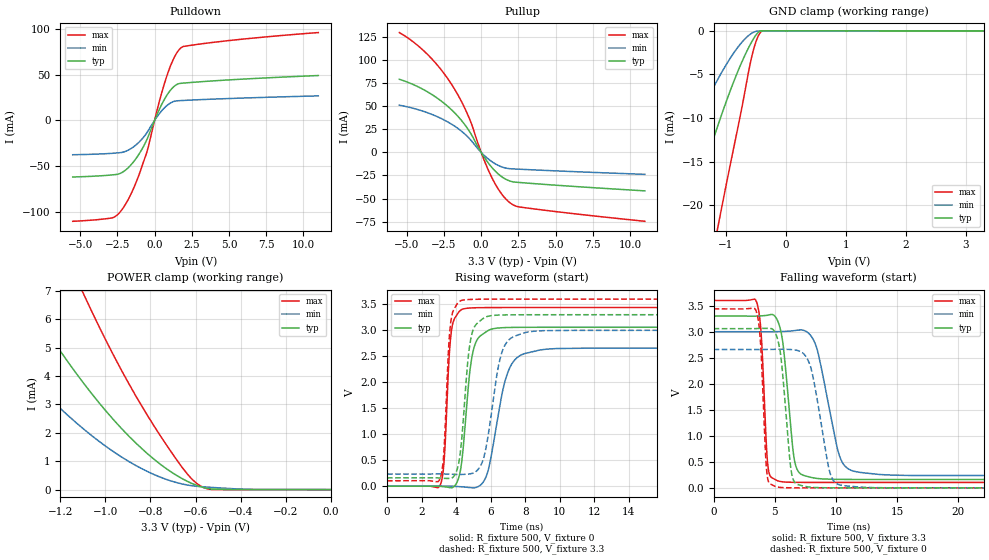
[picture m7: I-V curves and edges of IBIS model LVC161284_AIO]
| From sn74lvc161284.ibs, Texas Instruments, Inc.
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[Model]   LVC161284_AIO
Model_type  I/O
Vinl=0.8
Vinh=2.0
Enable   Active-Low
Vref =   0
Rref =   500
Cref =   50p
Vmeas =   1.5
| variable   typ   min   max
C_comp   7pF   NA   15pF
| C_pullup   4.48pF   2.95pF   5.26pF
| C_pulldown   4.78pF   2.73pF   7.37pF
| C_tri-state   3.06pF   2.68pF   3.49pF
[Temperature Range]   40   100   -40
| Ambient temperature   25   85   -40
[Voltage range]   3.3   3   3.6
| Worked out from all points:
|   slope of the pulldown table from 0 to 0.495 V, typ, clamps not added: 27.6 ohm
|   slope of the pullup table from 0 to 0.495 V, typ, clamps not added: 41.7 ohm
|   GND clamp passes 1 mA (typ) near -0.54 V on its own axis
|   POWER clamp passes 1 mA (typ) near -0.77 V on its own axis
|   rising waveform, R_fixture 500, V_fixture 0: 20-80 % time 523ps typ, 923ps min, 310ps max; typ from 0 V to 3.06 V
|   falling waveform, R_fixture 500, V_fixture 3.3: 20-80 % time 739ps typ, 1.41ns min, 417ps max; typ from 3.3 V to 0.161 V
|   rising waveform, R_fixture 500, V_fixture 3.3: 20-80 % time 482ps typ, 786ps min, 298ps max; typ from 0.161 V to 3.3 V
|   falling waveform, R_fixture 500, V_fixture 0: 20-80 % time 669ps typ, 1.16ns min, 393ps max; typ from 3.06 V to 0 V
[GND Clamp]
| LVC161284_AIO
|   Voltage   I(typ)   I(min)   I(max)
-5.5V     -124.6mA   -80.94mA   -210.5mA
-2.235V   -36.57mA   -22.18mA   -65.82mA
-1.66V    -22.55mA   -12.99mA   -42.47mA
-1.595V   -21.04mA   -12.01mA   -39.93mA
-1.35V    -15.52mA   -8.465mA   -30.56mA
-1.125V   -10.77mA   -5.487mA   -22.35mA
-1.095V   -10.16mA   -5.116mA   -21.29mA
-830mV    -5.215mA   -2.195mA   -12.23mA
-575mV    -1.378mA   -319uA     -3.275mA
-485mV    -388.3uA   -48.19uA   -1.058mA
-405mV    -426nA     -15.14uA   -79.63uA
3.3V      15.69pA    1.759uA    12.9pA
[POWER Clamp]
| LVC161284_AIO
|   Voltage   I(typ)   I(min)   I(max)
-5.5V     95.74mA    66.5mA     147.1mA
-1.67V    11.2mA     7.076mA    18.75mA
-1.63V    10.6mA     6.666mA    17.81mA
-1.375V   7.021mA    4.263mA    12.17mA
-1.34V    6.57mA     3.965mA    11.46mA
-1.095V   3.726mA    2.12mA     6.854mA
-960mV    2.424mA    1.312mA    4.669mA
-815mV    1.275mA    642.3uA    2.632mA
-660mV    389.4uA    200uA      789uA
-595mV    150.4uA    116.8uA    222.1uA
-525mV    17.62uA    75.98uA    163.3nA
-95.1fV   15.69pA    148.5pA    17.15pA
[Pulldown]
| LVC161284_AIO
|   Voltage   I(typ)   I(min)   I(max)
-5.5V     -61.78mA   -37.48mA   -110.1mA
-2.825V   -59.44mA   -35.9mA    -106.3mA
-2.43V    -58.53mA   -35.39mA   -102mA
-2V       -54.84mA   -34.05mA   -92.8mA
-1.3V     -42.78mA   -27.43mA   -69.93mA
-565mV    -22.58mA   -14.58mA   -36.9mA
355mV     13.3mA     8.102mA    22.85mA
925mV     29.88mA    17.45mA    53.24mA
1.375V    37.93mA    21.07mA    70.43mA
1.785V    40.5mA     21.65mA    79.37mA
4.84V     44.06mA    23.79mA    86.88mA
11V       48.99mA    26.77mA    95.88mA
[Pullup]
| LVC161284_AIO
|   Voltage   I(typ)   I(min)   I(max)
-5.5V     79.04mA    51.01mA    129.6mA
-3.635V   65.72mA    43.01mA    106.4mA
-2.785V   56.72mA    37.37mA    91.28mA
-2.015V   46.38mA    30.72mA    74.2mA
-1.415V   36.26mA    24.06mA    57.82mA
-890mV    25.17mA    16.58mA    40.26mA
105mV     -2.737mA   -1.728mA   -4.511mA
700mV     -15.99mA   -9.877mA   -26.74mA
1.32V     -25.66mA   -15.34mA   -43.8mA
1.935V    -31.04mA   -17.69mA   -54.52mA
2.56V     -32.58mA   -18.23mA   -59.08mA
11V       -41.67mA   -23.8mA    -74.59mA
[Ramp]
| LVC161284_AIO
| variable   typ   min   max
dV/dt_r   1.85/5.34E-10   1.61/9.33E-10   2.08/3.16E-10
dV/dt_f   1.90/7.52E-10   1.68/1.43E-09   2.11/4.28E-10
R_load = 500
[Rising Waveform]
| LVC161284_AIO
R_fixture =   500
C_fixture =   0
L_fixture =   0
V_fixture =   0
V_fixture_min = 0
V_fixture_max = 0
|   Time   V(typ)   V(min)   V(max)
0s        81.16pV    6.348nV    51.41pV
3.075ns   -2.658mV   1.301mV    19.49mV
3.31ns    -11.42mV   1.864mV    517.6mV
3.72ns    -30.24mV   -138.6uV   2.968V
4.47ns    965.6mV    -15.38mV   3.416V
4.85ns    2.349V     -28.33mV   3.43V
5.27ns    2.846V     -8.809mV   3.435V
7.085ns   3.054V     2.265V     3.438V
8.845ns   3.058V     2.621V     3.438V
50ns      3.059V     2.658V     3.438V
[Falling Waveform]
| LVC161284_AIO
R_fixture =   500
C_fixture =   0
L_fixture =   0
V_fixture =   3.3
V_fixture_min = 3
V_fixture_max = 3.6
|   Time   V(typ)   V(min)   V(max)
0s        3.3V       3V         3.6V
3.52ns    3.3V       2.999V     3.564V
3.88ns    3.304V     2.999V     2.97V
4.435ns   3.318V     2.999V     421.9mV
5.305ns   3.165V     3.002V     130.5mV
6.59ns    549.8mV    3.021V     106.3mV
7.48ns    230.8mV    3.015V     104.8mV
10.29ns   163.1mV    609.4mV    104.4mV
11.44ns   161.5mV    320.6mV    104.4mV
50ns      160.7mV    234.5mV    104.4mV
[Rising Waveform]
| LVC161284_AIO
R_fixture =   500
C_fixture =   0
L_fixture =   0
V_fixture =   3.3
V_fixture_min = 3
V_fixture_max = 3.6
|   Time   V(typ)   V(min)   V(max)
0s        160.7mV    234.5mV    104.4mV
3.055ns   157mV      235.5mV    132.3mV
3.275ns   151.3mV    235.1mV    583.6mV
3.69ns    151.4mV    231.3mV    3.158V
4.38ns    1.131V     226.9mV    3.581V
5.08ns    3.078V     265.7mV    3.596V
5.665ns   3.248V     636.9mV    3.599V
6.7ns     3.296V     2.621V     3.6V
8.155ns   3.3V       2.968V     3.6V
50ns      3.3V       3V         3.6V
[Falling Waveform]
| LVC161284_AIO
R_fixture =   500
C_fixture =   0
L_fixture =   0
V_fixture =   0
V_fixture_min = 0
V_fixture_max = 0
|   Time   V(typ)   V(min)   V(max)
0s        3.059V     2.658V     3.438V
3.48ns    3.06V      2.657V     3.394V
3.845ns   3.063V     2.658V     2.738V
4.365ns   3.064V     2.659V     262.1mV
5.125ns   2.93V      2.662V     21.09mV
6.33ns    338.1mV    2.657V     1.193mV
6.985ns   55.63mV    2.629V     387.3uV
7.93ns    12.93mV    2.318V     100.4uV
10.32ns   521.3uV    55.06mV    11.3uV
50ns      288nV      881.7nV    89.19nV
